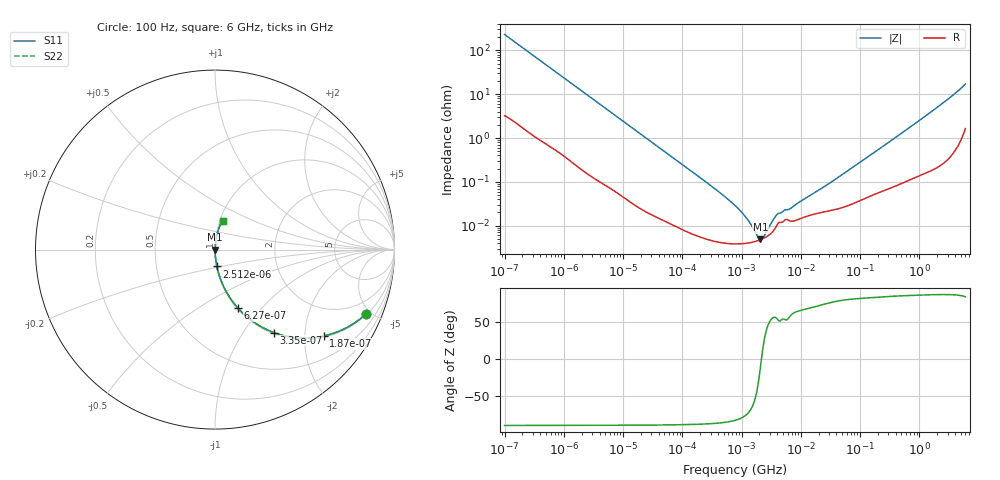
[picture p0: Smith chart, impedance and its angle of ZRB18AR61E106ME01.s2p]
!Murata Part Number: ZRB18AR61E106ME01
!These Parameters are Measured in Series Mode Connection
!Data Generated on Jun 10, 2025
!  o--ll--o
!Port1  Port2
!  o------o
!Operation Temp=25[degC], DC Bias Voltage=0[V]
!Freq. Start=100[Hz] Stop=6[GHz] 401[Steps]
# Hz S RI R 50
!Freq.(Hz) S11(Real) S11(Imag) S21(Real) S21(Imag) S12(Real) S12(Imag) S22(Real) S22(Imag)
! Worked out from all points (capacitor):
!   401 points, 100 Hz to 6 GHz, reference 50 ohm
!   read as one part in series: C = 6.87 uF near 109 Hz
!   lowest |Z| = 4.85 mohm at 2.074 MHz (marker M1)
!   series resonance near 2.16 MHz, so ESL is about 790 pH
!   S11 on the Smith chart (normalised r, x): 100 Hz: 1.06, -4.62; 187 Hz: 1.04, -2.48; 335 Hz: 1.02, -1.40; 627 Hz: 1.01, -0.75; 2.512 kHz: 1.00, -0.19; 6 GHz: 1.03, +0.34
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100  0.8386 -0.361  0.1614 0.361  0.1614 0.361  0.8386 -0.361
131  0.7549 -0.4229  0.2451 0.4229  0.2451 0.4229  0.7549 -0.4229
187  0.6053 -0.4815  0.3947 0.4815  0.3947 0.4815  0.6053 -0.4815
335  0.3298 -0.4628  0.6702 0.4628  0.6702 0.4628  0.3298 -0.4628
627  0.1272 -0.3253  0.8728 0.3253  0.8728 0.3253  0.1272 -0.3253
1026  0.0537 -0.2173  0.9463 0.2173  0.9463 0.2173  0.0537 -0.2173
2008  0.0156 -0.1165  0.9844 0.1165  0.9844 0.1165  0.0156 -0.1165
2512  0.0104 -0.0938  0.9896 0.0938  0.9896 0.0938  0.0104 -0.0938
7358  0.00167 -0.0327  0.9983 0.0327  0.9983 0.0327  0.00167 -0.0327
40335  0.000183 -0.00608  0.9998 0.00608  0.9998 0.00608  0.000183 -0.00608
316350  4.58e-05 -0.00078  1 0.00078  1 0.00078  4.58e-05 -0.00078
774597  3.83e-05 -0.000285  1 0.000285  1 0.000285  3.83e-05 -0.000285
1449809  4.12e-05 -9.59e-05  1 9.59e-05  1 9.59e-05  4.12e-05 -9.59e-05
1585629  4.24e-05 -7.35e-05  1 7.35e-05  1 7.35e-05  4.24e-05 -7.35e-05
2074311  4.76e-05 -9.5e-06  1 9.5e-06  1 9.5e-06  4.76e-05 -9.5e-06
2837864  5.94e-05 6.5e-05  0.9999 -6.5e-05  0.9999 -6.5e-05  5.94e-05 6.5e-05
4060267  0.000109 0.00015  0.9999 -0.00015  0.9999 -0.00015  0.000109 0.00015
6644369  0.000127 0.000209  0.9999 -0.000209  0.9999 -0.000209  0.000127 0.000209
1.555665e7  0.000178 0.000493  0.9998 -0.000493  0.9998 -0.000493  0.000178 0.000493
3.124326e8  0.000768 0.00813  0.9992 -0.00813  0.9992 -0.00813  0.000768 0.00813
1.95892e9  0.00444 0.0486  0.9956 -0.0486  0.9956 -0.0486  0.00444 0.0486
6e9  0.043 0.1605  0.957 -0.1605  0.957 -0.1605  0.043 0.1605
